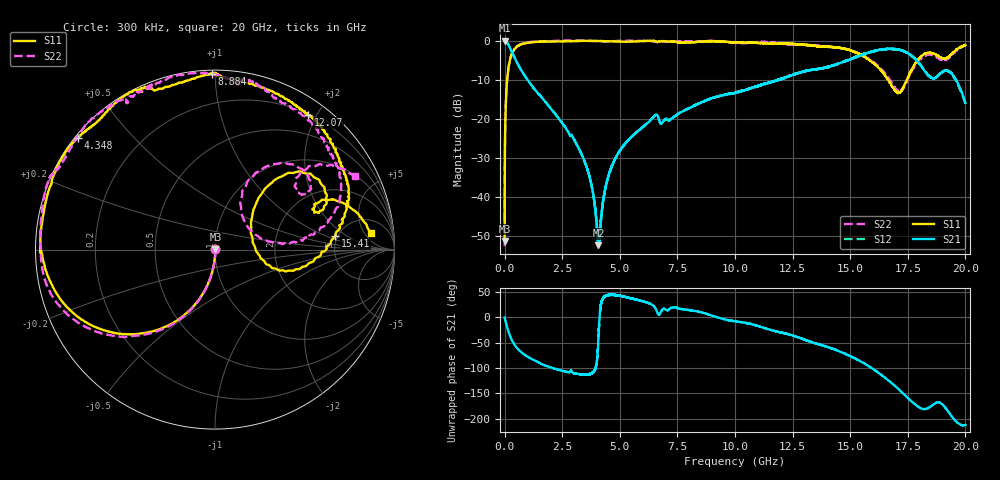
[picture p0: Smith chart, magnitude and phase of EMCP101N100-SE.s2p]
!EMCP101N100
!Johanson Technology Inc.
!www.johansontechnology.com
!Test Board Conditions:
!Substrate Type  RO4350B
!Substrate Thickness  10 mil
!Substrate Dk  3.66
!TL Type: GCPW
!TL Trace Width  20 mil
!TL Gap  10 mil
!PART MODE SINGLE ENDED (AKA BYPASS)
!DUT TOPOLOGY	SERIES-SHUNT
# MHz S  dB  R 50
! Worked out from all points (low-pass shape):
!   20001 points, 300 kHz to 20 GHz, reference 50 ohm
!   highest |S21| = -0.01 dB at 1.3 MHz (marker M1); lowest = -52.4 dB at 4.075 GHz (marker M2)
!   |S21| within 3 dB of the highest: start of sweep to 328.1 MHz; 15.82 GHz to 17.44 GHz (1.62 GHz wide, 9.74 % of centre)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
!   lowest |S11| = -51.3 dB at 300 kHz (marker M3), VSWR 1.01, Z = 50.2 + j0.146 ohm
!   |S11| at or under -10 dB: start of sweep to 110.9 MHz; 16.64476 GHz to 16.64672 GHz (1.952 MHz wide, 0.0117 % of centre); 16.65 GHz to 17.46 GHz (816.2 MHz wide, 4.79 % of centre)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
!   |S22| runs from -52.6 to 0.1 dB; largest |S21 - S12| = 0.02
!   S11 on the Smith chart (normalised r, x): 300 kHz: 1.00, +0.00; 4.348 GHz: 0.01, +0.36; 8.884 GHz: 0.02, +0.98; 12.07 GHz: 0.21, +1.89; 15.41 GHz: 4.73, +1.29; 20 GHz: 9, +7
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0.3  -51.28 32.1  -0.03 -0.2  -0.02 -0.1  -52.64 29.3
1.3  -48.32 -64.4  -0.01 -0.3  -0.01 -0.3  -47.97 -67.0
125.298  -9.07 -111.7  -0.63 -21.5  -0.62 -21.4  -9.03 -111.4
376.294  -2.65 -141.3  -3.62 -49.8  -3.60 -50.0  -2.60 -139.6
1148.283  -0.43 -173.5  -11.25 -81.4  -11.28 -81.3  -0.32 -170.3
3334.25  -0.06 151.2  -28.99 -112.8  -29.01 -112.7  0.00 155.3
3759.244  -0.05 145.6  -36.64 -111.5  -36.67 -110.6  -0.10 153.6
4075.239  -0.09 142.7  -52.42 -38.2  -52.09 -39.4  -0.14 151.6
4348.235  -0.14 140.7  -38.49 41.9  -38.53 41.6  -0.17 149.0
5099.224  -0.28 134.5  -27.38 42.3  -27.44 42.1  -0.05 138.4
6667.2  -0.29 114.9  -19.58 6.3  -19.54 5.9  -0.43 120.7
8884.167  -0.17 90.9  -14.94 5.6  -14.99 5.5  -0.08 103.7
10000.15  -0.44 85.5  -13.40 -7.6  -13.21 -7.4  -0.56 82.8
12074.12  -0.80 55.4  -9.72 -30.4  -9.54 -29.9  -0.81 69.2
13334.1  -1.27 38.5  -7.51 -48.9  -7.48 -49.3  -1.21 48.0
15407.07  -3.45 6.4  -3.90 -85.6  -3.73 -86.1  -3.40 15.8
16667.05  -10.24 -16.0  -2.10 -124.9  -2.17 -124.5  -9.56 6.6
17199.04  -13.05 25.9  -2.42 -145.9  -2.43 -145.1  -12.91 42.2
18043.03  -4.26 44.4  -6.20 -178.9  -6.11 -178.4  -4.69 55.0
18552.02  -3.19 26.6  -9.55 -174.4  -9.46 -174.9  -3.67 36.3
19342.01  -3.69 25.0  -8.06 168.1  -8.15 166.9  -4.00 41.5
20000  -1.16 6.0  -15.91 147.0  -16.18 148.6  -1.05 27.4
